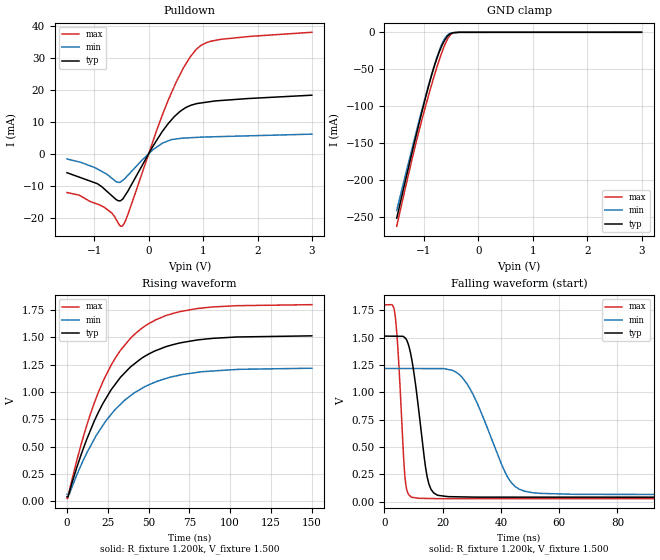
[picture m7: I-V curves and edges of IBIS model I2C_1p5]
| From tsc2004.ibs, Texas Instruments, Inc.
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| Model 1.5 V I2C
[Model]   I2C_1p5
Model_type   I/O_open_drain
Polarity   Non-Inverting
Enable   Active-Low
Vinl = 0.3
Vinh = 1.05
Vmeas = 0.8
Vref = 0.8
Cref = 15pF
Rref = 1200
|   typ   min   max
|   (nom PVT)   (Fast PVT)   (slow PVT)
|   Output High
C_comp   1.36799E-11   1.34922E-11   1.41279E-11
|   Output Low
|C_comp   1.36799E-11   1.32458E-11   1.41931E-11
| Where   nom PVT is  Nominal Process, 3.3V, 25C
|   Fast PVT is Strong Process, 3.6V, -40C
|   Slow PVT is Weak Process, 3.0V, 85C
|C_comp - from L-C Tank method, L = 1nH, peak frequency ~ 1.35GHz
[Model Spec]   | power 1.5, 1.2, 1.8 V
Vinl   0.3   0.24   0.54
Vinh   1.05   0.84   1.26
[Voltage Range]   1.5   1.2   1.8
[Temperature Range]   30   88   -40
|Ambient Temperature Range 27   85   -40
[Pullup Reference]   1.5   1.2   1.8
[Pulldown Reference]   0   0   0
[Power Clamp Reference]   1.5   1.2   1.8
[GND Clamp Reference]   0   0   0
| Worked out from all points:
|   slope of the pulldown table from 0 to 0.225 V, typ, clamps not added: 35.7 ohm
|   GND clamp passes 1 mA (typ) near -0.48 V on its own axis
|   falling waveform, R_fixture 1.200k, V_fixture 1.500: 20-80 % time 4.13ns typ, 10.7ns min, 2.13ns max; typ from 1.51 V to 0.042 V
|   rising waveform, R_fixture 1.200k, V_fixture 1.500: 20-80 % time 31.6ns typ, 33.2ns min, 30.1ns max; typ from 0.042 V to 1.51 V
[Pulldown]
|   Voltage   I(typ)   I(min)   I(max)
-1.5V     -5.989mA   -1.695mA   -12.18mA
-814.1mV  -11.08mA   -6.018mA   -16.83mA
-596.4mV  -14.39mA   -8.812mA   -20.61mA
-486.8mV  -14.38mA   -8.479mA   -22.68mA
-389.4mV  -11.94mA   -6.929mA   -19.37mA
78.97mV   2.312mA    1.198mA    3.884mA
357.8mV   9.361mA    3.967mA    16.65mA
633.3mV   13.84mA    4.823mA    26.64mA
874.4mV   15.58mA    5.047mA    32.59mA
1.048V    16.03mA    5.184mA    34.59mA
1.322V    16.58mA    5.308mA    35.69mA
2.995V    18.24mA    6.068mA    37.9mA
[GND Clamp]
|   Voltage   I(typ)   I(min)   I(max)
-1.5V     -252mA     -241.6mA   -263mA
-1.302V   -188.8mA   -181.9mA   -198.3mA
-1.151V   -142mA     -137.6mA   -151.3mA
-975.9mV  -90mA      -88mA      -101.7mA
-855.7mV  -57.29mA   -56.21mA   -70.13mA
-728.3mV  -28.45mA   -26.71mA   -39.6mA
-645.8mV  -14.42mA   -11.94mA   -22.3mA
-567.7mV  -5.373mA   -3.813mA   -9.225mA
-498.7mV  -1.394mA   -986.1uA   -2.427mA
-442.2mV  -479.3uA   -427.3uA   -486.1uA
-351mV    -26uA      -28.52uA   -17.64uA
2.995V    0A         0A         0A
[POWER Clamp]
|   SCR cell for ESD function. Effects occurr above VDD x 2
|   Voltage   I(typ)   I(min)   I(max)
-1.5V     0A         0A         0A
0V        0A         0A         0A
3V        0A         0A         0A
[Ramp]
R_load = 1200
|   typ   min   max
dV/dt_r   0.87508/3.15815e-008  0.682162/3.31859e-008   1.06212/2.9979e-008
dV/dt_f   0.87508/4.11491e-009  0.682162/1.06879e-008   1.06212/2.12568e-009
[Falling Waveform]
R_fixture = 1.200k
V_fixture = 1.500
V_fixture_min = 1.200
V_fixture_max = 1.800
C_fixture = 0.000
|  time   V(typ)   V(min)   V(max)
0s        1.514V     1.218V     1.799V
3.626ns   1.513V     1.218V     1.707V
7.01ns    1.498V     1.218V     233.7mV
9.2ns     1.323V     1.218V     44.02mV
14.63ns   231.3mV    1.217V     31.05mV
18.24ns   60.95mV    1.217V     29.39mV
28.62ns   44.33mV    1.066V     29.36mV
42.13ns   42.99mV    232.6mV    29.31mV
47.98ns   42.94mV    97.95mV    29.29mV
150ns     42.06mV    64.93mV    28.95mV
[Rising Waveform]
R_fixture = 1.200k
V_fixture = 1.500
V_fixture_min = 1.200
V_fixture_max = 1.800
C_fixture = 0.000
|  time   V(typ)   V(min)   V(max)
0s        42.06mV    64.93mV    28.95mV
399.4ps   42.15mV    65.86mV    25.42mV
1.461ns   86.18mV    68.35mV    100mV
11.51ns   545.7mV    424.4mV    667.6mV
21.68ns   886.8mV    689mV      1.085V
32.89ns   1.137V     890.5mV    1.384V
45.15ns   1.303V     1.027V     1.575V
59.98ns   1.412V     1.121V     1.696V
78.78ns   1.474V     1.178V     1.761V
150ns     1.514V     1.218V     1.799V
